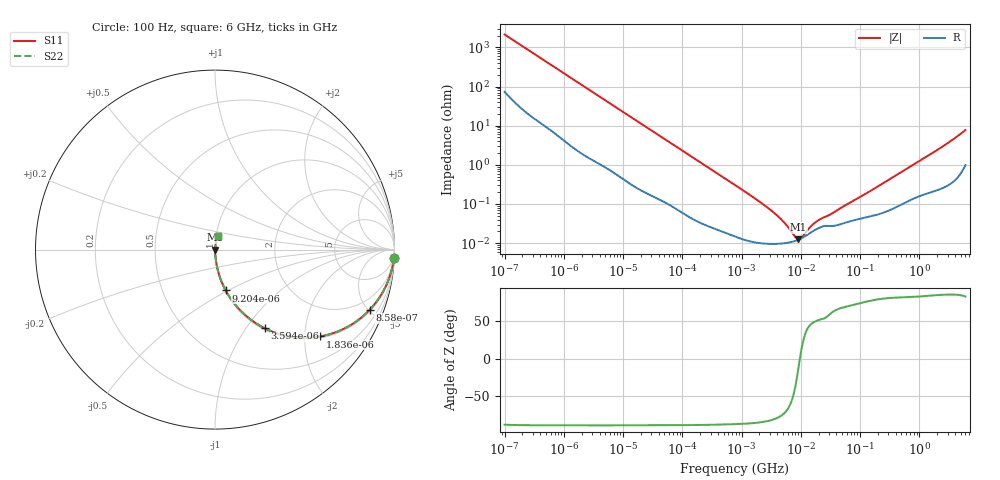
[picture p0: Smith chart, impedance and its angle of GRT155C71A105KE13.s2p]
!Murata Part Number: GRT155C71A105KE13
!These Parameters are Measured in Series Mode Connection
!Data Generated on Jun 19, 2026
!  o--ll--o
!Port1  Port2
!  o------o
!Operation Temp=25[degC], DC Bias Voltage=0[V]
!Freq. Start=100[Hz] Stop=6[GHz] 401[Steps]
# Hz S RI R 50
!Freq.(Hz) S11(Real) S11(Imag) S21(Real) S21(Imag) S12(Real) S12(Imag) S22(Real) S22(Imag)
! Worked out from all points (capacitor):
!   401 points, 100 Hz to 6 GHz, reference 50 ohm
!   read as one part in series: C = 745 nF near 109 Hz
!   lowest |Z| = 12.6 mohm at 9.09 MHz (marker M1)
!   series resonance near 9.651 MHz, so ESL is about 370 pH
!   S11 on the Smith chart (normalised r, x): 100 Hz: 2, -43; 858 Hz: 1.10, -5.08; 1.836 kHz: 1.04, -2.39; 3.594 kHz: 1.02, -1.23; 9.204 kHz: 1.01, -0.49; 6 GHz: 1.02, +0.15
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100  0.9962 -0.0467  0.0038 0.0467  0.0038 0.0467  0.9962 -0.0467
320  0.9753 -0.1446  0.0247 0.1446  0.0247 0.1446  0.9753 -0.1446
858  0.8611 -0.3361  0.1389 0.3361  0.1389 0.3361  0.8611 -0.3361
1836  0.5871 -0.4837  0.4129 0.4837  0.4129 0.4837  0.5871 -0.4837
2008  0.5443 -0.4893  0.4557 0.4893  0.4557 0.4893  0.5443 -0.4893
3594  0.2782 -0.4389  0.7218 0.4389  0.7218 0.4389  0.2782 -0.4389
5625  0.14 -0.3374  0.86 0.3374  0.86 0.3374  0.14 -0.3374
9204  0.0598 -0.2276  0.9402 0.2276  0.9402 0.2276  0.0598 -0.2276
18016  0.0177 -0.1226  0.9823 0.1226  0.9823 0.1226  0.0177 -0.1226
40335  0.00448 -0.0561  0.9955 0.0561  0.9955 0.0561  0.00448 -0.0561
774597  0.000157 -0.00305  0.9998 0.00305  0.9998 0.00305  0.000157 -0.00305
3549919  9.62e-05 -0.000585  0.9999 0.000585  0.9999 0.000585  9.62e-05 -0.000585
5311619  9.99e-05 -0.000315  0.9999 0.000315  0.9999 0.000315  9.99e-05 -0.000315
7947587  0.000114 -9.59e-05  0.9999 9.59e-05  0.9999 9.59e-05  0.000114 -9.59e-05
9090158  0.000123 -2.91e-05  0.9999 2.91e-05  0.9999 2.91e-05  0.000123 -2.91e-05
1.039699e7  0.000135 3.6e-05  0.9999 -3.6e-05  0.9999 -3.6e-05  0.000135 3.6e-05
1.555665e7  0.000198 0.000213  0.9998 -0.000213  0.9998 -0.000213  0.000198 0.000213
2.128304e7  0.000253 0.000325  0.9997 -0.000325  0.9997 -0.000325  0.000253 0.000325
3.184506e7  0.000273 0.000473  0.9997 -0.000473  0.9997 -0.000473  0.000273 0.000473
3.124326e8  0.000706 0.0042  0.9993 -0.0042  0.9993 -0.0042  0.000706 0.0042
1.873145e9  0.00266 0.0221  0.9973 -0.0221  0.9973 -0.0221  0.00266 0.0221
6e9  0.0154 0.0747  0.9846 -0.0747  0.9846 -0.0747  0.0154 0.0747
